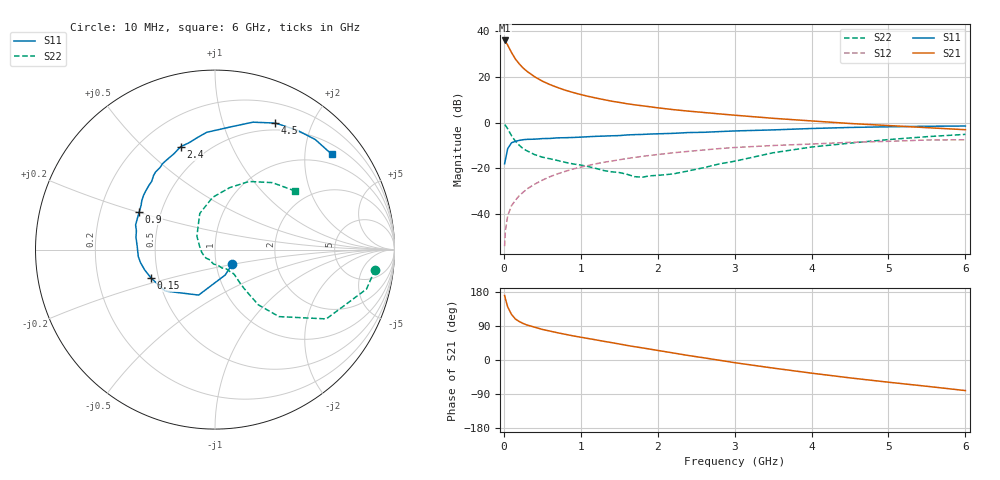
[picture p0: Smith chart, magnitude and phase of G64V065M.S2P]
! SIEMENS Small Signal Semiconductors
! BFG193
! Si NPN RF Bipolar Junction Transistor in SOT223
! VCE = 4 V  IC = 65 mA
! Common Emitter S-Parameters:  August  1996
# GHz  S  MA  R  50
!  f  S11  S21  S12  S22
! GHz  MAG  ANG  MAG  ANG  MAG  ANG  MAG  ANG
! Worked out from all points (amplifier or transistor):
!   36 points, 10 MHz to 6 GHz, reference 50 ohm
!   highest |S21| = 35.8 dB at 10 MHz (marker M1)
!   |S21| within 3 dB of that: start of sweep to 64.72 MHz
!   unconditionally stable (mu >= 1): 362.2 MHz to 2.339 GHz
!   at 250 MHz: K = 0.95, MSG = 27.1 dB, |S12| = -30.5 dB
!   at 1.4 GHz: K = 1.05, MAG = 11.7 dB, |S12| = -16.8 dB
!   at 6 GHz: K = 0.90, MSG = 2.2 dB, |S12| = -7.5 dB
!   S11 on the Smith chart (normalised r, x): 10 MHz: 1.19, -0.20; 150 MHz: 0.46, -0.17; 900 MHz: 0.38, +0.20; 2.4 GHz: 0.36, +0.66; 4.5 GHz: 0.42, +1.50; 6 GHz: 0.73, +2.62
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0.01  0.1258 -40.7  61.91 170.3  0.002 88.0  0.8988 -7.1
0.02  0.1527 -68.2  59.3 162.0  0.0043 74.6  0.8723 -14.6
0.05  0.2693 -109.8  48.91 140.0  0.0092 69.4  0.7306 -31.9
0.1  0.3612 -140.3  33.7 120.2  0.0154 69.1  0.5166 -46.3
0.15  0.3896 -155.9  24.4 108.2  0.02 68.2  0.3903 -51.9
0.2  0.4071 -163.6  19.12 101.6  0.0253 69.6  0.3202 -52.6
0.25  0.4213 -170.0  15.55 96.4  0.03 70.5  0.2693 -53.2
0.3  0.4292 -174.9  13.15 92.4  0.0354 71.0  0.2415 -53.3
0.4  0.4334 178.0  9.996 86.6  0.0451 71.1  0.1995 -52.7
0.5  0.4461 170.9  8.014 80.7  0.0551 69.6  0.1753 -52.1
0.6  0.4499 166.7  6.728 76.3  0.0658 68.4  0.1615 -53.3
0.7  0.463 162.8  5.799 71.8  0.0759 67.2  0.1482 -55.8
0.9  0.4718 153.4  4.525 63.7  0.0968 63.3  0.1249 -59.4
1.1  0.4904 146.3  3.719 56.6  0.116 59.8  0.1092 -69.3
1.3  0.5061 139.5  3.16 49.3  0.1356 55.7  0.0895 -78.4
1.6  0.5361 129.7  2.575 38.5  0.1639 48.7  0.0743 -102.7
2.2  0.5809 113.2  1.916 18.6  0.2183 35.1  0.0755 -168.0
2.4  0.6044 108.5  1.775 11.8  0.2348 30.8  0.088 167.6
3.5  0.6906 82.4  1.237 -21.3  0.3151 3.6  0.2187 112.8
4.5  0.781 64.5  0.953 -47.2  0.37 -16.6  0.3554 76.5
5.5  0.8295 47.7  0.773 -69.4  0.4154 -40.0  0.4913 49.4
6  0.8394 39.3  0.697 -80.7  0.4206 -53.5  0.5517 36.4
